| TEXAS INSTRUMENTS INCORPORATED
| Standard Linear and Logic Group
| IBIS Model of SN74LVC541A
| OCTAL BUFFERS/DRIVERS WITH 3-STATE OUTPUTS
| This file contains package information for the following:
|  SSOP 20-pin (DB) package as [Component] LVC541A_DB
|  TVSOP 20-pin (DGV) package as [Component] LVC541A_DGV
|  SOIC 20-pin (DW) package as [Component] LVC541A_DW
|  SOP 20-pin (NS) package as [Component] LVC541A_NS
|  QFN 20-pin (RGY) package as [Component] LVC541A_RGY
|  TSSOP 20-pin (PW) package as [Component] LVC541A_PW
| This device can be powered at the following Vccs:
|  1.8 volt Vcc
|  2.5 volt Vcc
|  3.3 volt Vcc
| This file provides unique models under the [Model Selector] for each Vcc.
| For operation at a specific Vcc, select the appropriate model after each
| [Model Selector] keyword.
[IBIS Ver]   3.2
[Comment char]  |_char
[File Name]   sn74lvc541a.ibs
[File Rev]   1.1 | e_die
[Date]   April 15, 2004
[Source]   Data created from TI-SPICE simulations at TI-SLL.
[Notes]   The following is an IBIS list for the LVC541A.
   Please contact sllibis@ti.com with questions and
   comments concerning SLL IBIS models.
   This IBIS model is created from a BA (back annotated netlist)
   - FILE REV HISTORY
   - 1.1 Release IBIS file on 04/15/04
   - Power clamp data deleted as there is no power-clamp diode.
   - Due to the fact that the Device is 5-V Input/Output
   tolarent, the output model has some Non-Monotonic Warnings.
   - 1.2 Release IBIS file on 5/21/20
   - Added 20-pin TSSOP package (PW)
[Disclaimer] Property of Texas Instruments Incorporated.  Unauthorized
   reproduction and/or distribution is strictly prohibited.
   This product is protected under copyright law.
   Created  2004, (C) Copyright  2004, Texas Instruments
   Incorporated, All Rights Reserved
   UNLESS THERE IS A SIGNED, WRITTEN AGREEMENT TO THE
   CONTRARY, TEXAS INSTRUMENTS (TI) IS PROVIDING THE IBIS
   MODELS  AND WITHOUT ANY WARRANTY, EXPRESSED OR
   IMPLIED.  TI assumes no liability for:
   1) the accuracy of the IBIS models provided to your
   company;
   2) the proper functioning of these IBIS Models in your
   design or for any resulting applications; or
   3) infringement of patents, copyrights or intellectual
   property rights resulting from your use of these IBIS
   models.
   TI provides IBIS Models as a service to our customers.
   You and your company shall not distribute, sell or give
   these models to anyone else without prior written
   permission from TI.
   TI reserves the right to make changes to our products or
   to discontinue any semiconductor product or service
   without notice, and advises our customers to obtain the
   latest version of relevant information to verify, before
   placing orders, that the information being relied on is
   current.
   Please be aware that your receipt and use of the IBIS
   information provided shall serve as acceptance of these
   terms and conditions.  If you do not accept these terms,
   you should return or destroy the IBIS models and any
   other accompanying information immediately.
| Component LVC541A_DB 20-pin SSOP
[Component]   LVC541A_DB
[Manufacturer]   Texas Instruments, Inc.
[Package]
|   typ   min   max
R_pkg   4.000e-02   3.500e-02   5.100e-02
L_pkg   3.495e-09   3.035e-09   4.314e-09
C_pkg   4.200e-13   3.460e-13   5.020e-13
[Pin]   signal_name   model_name   R_pin   L_pin   C_pin
1   NOE1   LVC541A_NOE   4.900e-02   4.310e-09   5.020e-13
2   A1   LVC541A_IN   4.800e-02   3.903e-09   4.870e-13
3   A2   LVC541A_IN   3.500e-02   3.189e-09   3.960e-13
4   A3   LVC541A_IN   3.500e-02   3.036e-09   3.470e-13
5   A4   LVC541A_IN   3.500e-02   3.035e-09   3.670e-13
6   A5   LVC541A_IN   3.500e-02   3.035e-09   3.670e-13
7   A6   LVC541A_IN   3.500e-02   3.036e-09   3.470e-13
8   A7   LVC541A_IN   3.500e-02   3.189e-09   3.970e-13
9   A8   LVC541A_IN   4.700e-02   3.899e-09   4.880e-13
10   GND   GND   5.100e-02   4.314e-09   5.000e-13
11   Y8   LVC541A_OUT   5.100e-02   4.314e-09   5.000e-13
12   Y7   LVC541A_OUT   4.700e-02   3.899e-09   4.880e-13
13   Y6   LVC541A_OUT   3.500e-02   3.189e-09   3.970e-13
14   Y5   LVC541A_OUT   3.500e-02   3.036e-09   3.460e-13
15   Y4   LVC541A_OUT   3.500e-02   3.035e-09   3.670e-13
16   Y3   LVC541A_OUT   3.500e-02   3.035e-09   3.670e-13
17   Y2   LVC541A_OUT   3.500e-02   3.036e-09   3.460e-13
18   Y1   LVC541A_OUT   3.500e-02   3.189e-09   3.970e-13
19   NOE2   LVC541A_NOE   4.700e-02   3.899e-09   4.880e-13
20   VCC   POWER   5.100e-02   4.314e-09   5.020e-13
| Component LVC541A_DGV 20-pin TVSOP
[Component]   LVC541A_DGV
[Manufacturer]   Texas Instruments, Inc.
[Package]
|   typ   min   max
R_pkg   4.400e-02   3.800e-02   4.800e-02
L_pkg   2.561e-09   2.236e-09   2.961e-09
C_pkg   3.420e-13   2.640e-13   4.460e-13
[Pin]   signal_name   model_name   R_pin   L_pin   C_pin
1   NOE1   LVC541A_NOE   4.400e-02   2.935e-09   4.170e-13
2   A1   LVC541A_IN   4.200e-02   2.869e-09   4.460e-13
3   A2   LVC541A_IN   4.300e-02   2.399e-09   3.160e-13
4   A3   LVC541A_IN   4.400e-02   2.236e-09   2.650e-13
5   A4   LVC541A_IN   4.600e-02   2.278e-09   2.640e-13
6   A5   LVC541A_IN   4.500e-02   2.274e-09   2.640e-13
7   A6   LVC541A_IN   4.400e-02   2.285e-09   2.690e-13
8   A7   LVC541A_IN   4.300e-02   2.452e-09   3.200e-13
9   A8   LVC541A_IN   4.400e-02   2.900e-09   4.460e-13
10   GND   GND   4.400e-02   2.961e-09   4.180e-13
11   Y8   LVC541A_OUT   4.500e-02   2.954e-09   4.180e-13
12   Y7   LVC541A_OUT   4.200e-02   2.847e-09   4.430e-13
13   Y6   LVC541A_OUT   4.500e-02   2.453e-09   3.190e-13
14   Y5   LVC541A_OUT   4.500e-02   2.297e-09   2.690e-13
15   Y4   LVC541A_OUT   4.800e-02   2.334e-09   2.680e-13
16   Y3   LVC541A_OUT   4.800e-02   2.335e-09   2.670e-13
17   Y2   LVC541A_OUT   4.600e-02   2.299e-09   2.680e-13
18   Y1   LVC541A_OUT   4.600e-02   2.457e-09   3.200e-13
19   NOE2   LVC541A_NOE   4.300e-02   2.848e-09   4.410e-13
20   VCC   POWER   3.800e-02   2.812e-09   4.080e-13
| Component LVC541A_DW 20-pin SOIC
[Component]   LVC541A_DW
[Manufacturer]   Texas Instruments, Inc.
[Package]
|   typ   min   max
R_pkg   3.800e-02   3.300e-02   4.500e-02
L_pkg   5.012e-09   4.110e-09   6.349e-09
C_pkg   7.170e-13   5.300e-13   8.680e-13
[Pin]   signal_name   model_name   R_pin   L_pin   C_pin
1   NOE1   LVC541A_NOE   4.200e-02   6.336e-09   8.650e-13
2   A1   LVC541A_IN   4.300e-02   5.542e-09   8.670e-13
3   A2   LVC541A_IN   3.400e-02   4.714e-09   7.320e-13
4   A3   LVC541A_IN   3.400e-02   4.377e-09   5.910e-13
5   A4   LVC541A_IN   3.600e-02   4.130e-09   5.330e-13
6   A5   LVC541A_IN   3.500e-02   4.111e-09   5.300e-13
7   A6   LVC541A_IN   3.400e-02   4.284e-09   5.830e-13
8   A7   LVC541A_IN   3.400e-02   4.634e-09   7.260e-13
9   A8   LVC541A_IN   4.000e-02   5.518e-09   8.650e-13
10   GND   GND   4.300e-02   6.349e-09   8.660e-13
11   Y8   LVC541A_OUT   4.100e-02   6.281e-09   8.610e-13
12   Y7   LVC541A_OUT   4.500e-02   5.561e-09   8.680e-13
13   Y6   LVC541A_OUT   3.300e-02   4.778e-09   7.420e-13
14   Y5   LVC541A_OUT   3.500e-02   4.414e-09   5.960e-13
15   Y4   LVC541A_OUT   3.500e-02   4.110e-09   5.330e-13
16   Y3   LVC541A_OUT   3.600e-02   4.130e-09   5.330e-13
17   Y2   LVC541A_OUT   3.400e-02   4.377e-09   5.910e-13
18   Y1   LVC541A_OUT   3.400e-02   4.714e-09   7.310e-13
19   NOE2   LVC541A_NOE   4.300e-02   5.569e-09   8.680e-13
20   VCC   POWER   4.200e-02   6.308e-09   8.640e-13
| Component LVC541A_NS 20-pin SOP
[Component]   LVC541A_NS
[Manufacturer]   Texas Instruments, Inc.
[Package]
|   typ   min   max
R_pkg   4.400e-02   2.900e-02   5.800e-02
L_pkg   3.666e-09   2.317e-09   5.115e-09
C_pkg   5.480e-13   3.160e-13   7.250e-13
[Pin]   signal_name   model_name   R_pin   L_pin   C_pin
1   NOE1   LVC541A_NOE   5.800e-02   5.115e-09   7.250e-13
2   A1   LVC541A_IN   5.300e-02   4.591e-09   7.240e-13
3   A2   LVC541A_IN   4.900e-02   3.754e-09   5.720e-13
4   A3   LVC541A_IN   2.900e-02   2.549e-09   3.880e-13
5   A4   LVC541A_IN   3.100e-02   2.317e-09   3.160e-13
6   A5   LVC541A_IN   3.100e-02   2.317e-09   3.160e-13
7   A6   LVC541A_IN   2.900e-02   2.556e-09   3.990e-13
8   A7   LVC541A_IN   4.900e-02   3.754e-09   5.790e-13
9   A8   LVC541A_IN   5.300e-02   4.591e-09   7.240e-13
10   GND   GND   5.800e-02   5.115e-09   7.250e-13
11   Y8   LVC541A_OUT   5.800e-02   5.115e-09   7.250e-13
12   Y7   LVC541A_OUT   5.300e-02   4.591e-09   7.240e-13
13   Y6   LVC541A_OUT   4.900e-02   3.754e-09   5.790e-13
14   Y5   LVC541A_OUT   2.900e-02   2.557e-09   3.990e-13
15   Y4   LVC541A_OUT   3.100e-02   2.317e-09   3.160e-13
16   Y3   LVC541A_OUT   3.100e-02   2.317e-09   3.160e-13
17   Y2   LVC541A_OUT   2.900e-02   2.557e-09   3.990e-13
18   Y1   LVC541A_OUT   4.900e-02   3.754e-09   5.790e-13
19   NOE2   LVC541A_NOE   5.300e-02   4.591e-09   7.240e-13
20   VCC   POWER   5.800e-02   5.115e-09   7.250e-13
| Component LVC541A_RGY 20-pin QFN
[Component]   LVC541A_RGY
[Manufacturer]   Texas Instruments, Inc.
[Package]
|   typ   min   max
R_pkg   4.600e-02   3.500e-02   5.800e-02
L_pkg   1.036e-09   7.930e-10   1.295e-09
C_pkg   3.410e-13   3.300e-13   3.540e-13
[Pin]   signal_name   model_name   R_pin   L_pin   C_pin
1   NOE1   LVC541A_NOE   5.300e-02   1.181e-09   3.330e-13
2   A1   LVC541A_IN   5.800e-02   1.285e-09   3.520e-13
3   A2   LVC541A_IN   4.600e-02   1.020e-09   3.420e-13
4   A3   LVC541A_IN   3.900e-02   8.780e-10   3.300e-13
5   A4   LVC541A_IN   3.500e-02   7.950e-10   3.340e-13
6   A5   LVC541A_IN   3.500e-02   7.930e-10   3.340e-13
7   A6   LVC541A_IN   3.900e-02   8.730e-10   3.300e-13
8   A7   LVC541A_IN   4.500e-02   1.014e-09   3.420e-13
9   A8   LVC541A_IN   5.800e-02   1.285e-09   3.520e-13
10   GND   GND   5.600e-02   1.244e-09   3.490e-13
11   Y8   LVC541A_OUT   5.300e-02   1.179e-09   3.450e-13
12   Y7   LVC541A_OUT   5.800e-02   1.295e-09   3.520e-13
13   Y6   LVC541A_OUT   4.700e-02   1.038e-09   3.440e-13
14   Y5   LVC541A_OUT   4.000e-02   8.880e-10   3.330e-13
15   Y4   LVC541A_OUT   3.500e-02   7.980e-10   3.380e-13
16   Y3   LVC541A_OUT   3.500e-02   7.940e-10   3.370e-13
17   Y2   LVC541A_OUT   3.900e-02   8.800e-10   3.310e-13
18   Y1   LVC541A_OUT   4.600e-02   1.027e-09   3.430e-13
19   NOE2   LVC541A_NOE   5.800e-02   1.295e-09   3.540e-13
20   VCC   POWER   5.200e-02   1.169e-09   3.340e-13
| Component LVC541A_PW 20-pin TSSOP
[Component]   LVC541A_PW
[Manufacturer]   Texas Instruments, Inc.
[Package]
|   typ   min   max
R_pkg   5.000e-02   4.200e-02   6.000e-02
L_pkg   2.802e-09   2.248e-09   3.553e-09
C_pkg   3.170e-13   2.020e-13   4.430e-13
[Pin]   signal_name   model_name   R_pin   L_pin   C_pin
1   NOE1   LVC541A_NOE   5.500e-02   3.461e-09   4.400e-13
2   A1   LVC541A_IN   5.500e-02   3.150e-09   4.010e-13
3   A2   LVC541A_IN   4.200e-02   2.619e-09   3.020e-13
4   A3   LVC541A_IN   4.500e-02   2.273e-09   2.020e-13
5   A4   LVC541A_IN   4.500e-02   2.248e-09   2.240e-13
6   A5   LVC541A_IN   4.500e-02   2.273e-09   2.260e-13
7   A6   LVC541A_IN   4.400e-02   2.323e-09   2.050e-13
8   A7   LVC541A_IN   4.600e-02   2.704e-09   3.070e-13
9   A8   LVC541A_IN   6.000e-02   3.265e-09   4.110e-13
10   GND   GND   5.700e-02   3.506e-09   4.360e-13
11   Y8   LVC541A_OUT   5.800e-02   3.553e-09   4.370e-13
12   Y7   LVC541A_OUT   5.800e-02   3.193e-09   4.050e-13
13   Y6   LVC541A_OUT   4.200e-02   2.704e-09   3.110e-13
14   Y5   LVC541A_OUT   4.600e-02   2.392e-09   2.100e-13
15   Y4   LVC541A_OUT   4.700e-02   2.334e-09   2.290e-13
16   Y3   LVC541A_OUT   4.700e-02   2.300e-09   2.270e-13
17   Y2   LVC541A_OUT   4.700e-02   2.349e-09   2.070e-13
18   Y1   LVC541A_OUT   4.500e-02   2.677e-09   3.060e-13
19   NOE2   LVC541A_NOE   6.000e-02   3.235e-09   4.060e-13
20   VCC   POWER   5.600e-02   3.487e-09   4.430e-13
| Model LVC541A_NOE
[Model Selector]   LVC541A_NOE
LVC541A_NOE_18   1.8 volt Vcc
LVC541A_NOE_25   2.5 volt Vcc
LVC541A_NOE_33   3.3 volt Vcc
| Model LVC541A_IN
[Model Selector]   LVC541A_IN
LVC541A_IN_18   1.8 volt Vcc
LVC541A_IN_25   2.5 volt Vcc
LVC541A_IN_33   3.3 volt Vcc
| Model LVC541A_OUT
[Model Selector]   LVC541A_OUT
LVC541A_OUT_18   1.8 volt Vcc
LVC541A_OUT_25   2.5 volt Vcc
LVC541A_OUT_33   3.3 volt Vcc
| Models and submodels in the file (9): LVC541A_NOE_18 (Input), LVC541A_NOE_25 (Input), LVC541A_NOE_33 (Input), LVC541A_IN_18 (Input), LVC541A_IN_25 (Input), LVC541A_IN_33 (Input), LVC541A_OUT_18 (3-state), LVC541A_OUT_25 (3-state), LVC541A_OUT_33 (3-state)
